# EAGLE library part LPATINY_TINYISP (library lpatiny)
CONNECTOR
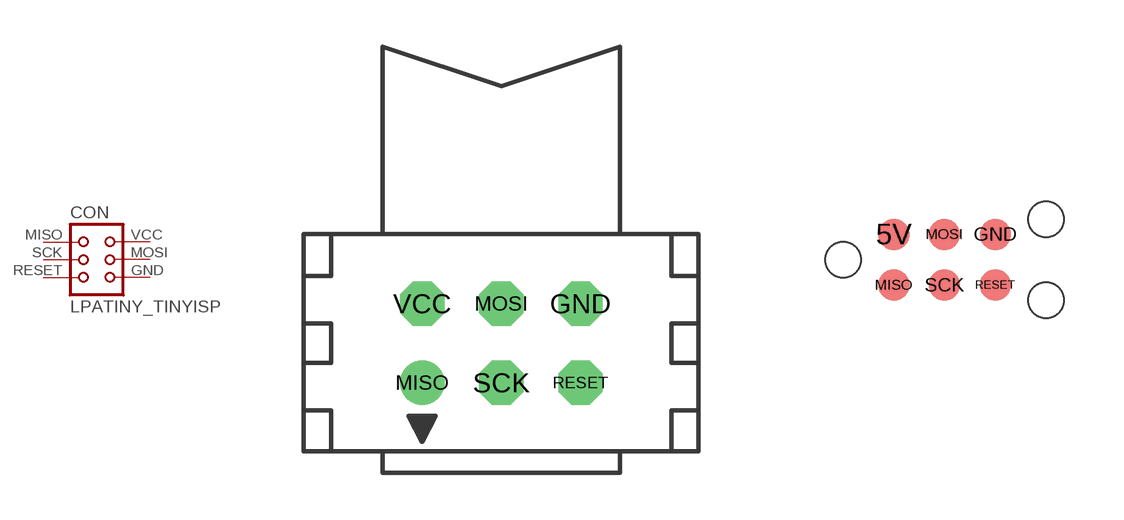
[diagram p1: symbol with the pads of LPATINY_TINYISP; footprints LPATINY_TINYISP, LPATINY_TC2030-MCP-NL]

Designator prefix CON

## LPATINY_TINYISP (OC_FARNELL: unknown; OC_NEWARK: unknown)  [LPATINY_TINYISP]
GND  GND  pas
MISO  MISO  pas
MOSI  MOSI  pas
RESET  RESET  pas
SCK  SCK  pas
VCC  VCC  pas

## LPATINY_TINYISPT  [LPATINY_TC2030-MCP-NL]
5V  VCC  pas
GND  GND  pas
MISO  MISO  pas
MOSI  MOSI  pas
RESET  RESET  pas
SCK  SCK  pas

## LPATINY_TINYISPTAG  [LPATINY_TC2030-MCP]
Pads as for LPATINY_TC2030-MCP-NL

## Footprint LPATINY_TINYISP (pad centres in mm)
CONNECTOR
drill 0.914 octagon: GND 2.54,1.27; MOSI 0,1.27; RESET 2.54,-1.27; SCK 0,-1.27; VCC -2.54,1.27
drill 0.914: MISO -2.54,-1.27

## Footprint LPATINY_TC2030-MCP-NL (pad centres in mm)
TAG-CONNECT ICSP Connector Manufacturer: Tag-Connect Cable for easy In-Circuit Serial Programming. Designed for Microchip ICD2, suitable for many others. PADDescription 1MCLR/Vpp 2Vdd 3GND 4PGD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
smd 0.787 x 0.787: 5V 1.27,0.635; GND 3.81,0.635; MISO 1.27,-0.635; MOSI 2.54,0.635; RESET 3.81,-0.635; SCK 2.54,-0.635
hole 0.889 at 0,0
hole 0.889 at 5.08,-1.016
hole 0.889 at 5.08,1.016

## Footprint LPATINY_TC2030-MCP (pad centres in mm)
TAG-CONNECT ICSP Connector - Legged version Manufacturer: Tag-Connect Cable for easy In-Circuit Serial Programming. Designed for Microchip ICD2, suitable for many others. NOTE: Eagle's default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
smd 0.787 x 0.787: 5V 1.27,0.635; GND 3.81,0.635; MISO 1.27,-0.635; MOSI 2.54,0.635; RESET 3.81,-0.635; SCK 2.54,-0.635
hole 0.889 at 0,0
hole 0.889 at 5.08,-1.016
hole 0.889 at 5.08,1.016
hole 2.375 at 0,2.54
hole 2.375 at 0,-2.54
hole 2.375 at 3.175,-2.54
hole 2.375 at 3.175,2.54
